(* Logix 5000 DataType export CTT2Command; software revision 32.01 *)

TYPE CTT2Command :
STRUCT
   Address : SINT;   // 1-31=1A-31A or 32-62= 31B-62B
   Command : SINT;   // 18=Read Venddor Specific Object
   Object : SINT;
   Length : SINT;
END_STRUCT
END_TYPE
